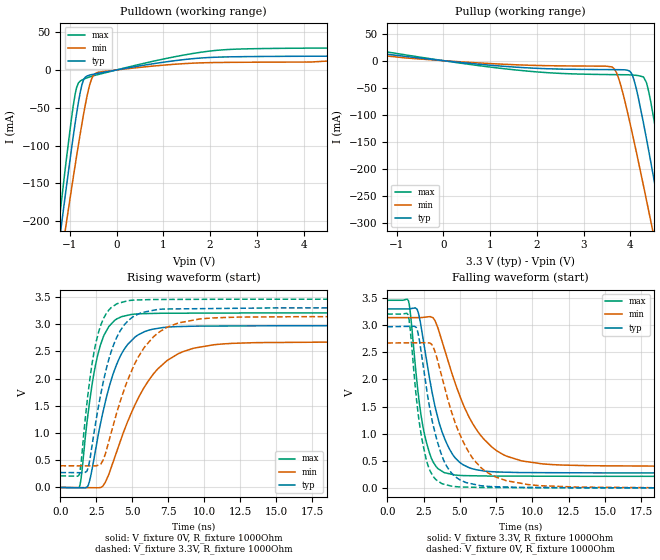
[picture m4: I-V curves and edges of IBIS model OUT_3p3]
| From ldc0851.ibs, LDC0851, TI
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|   Model
[Model]   OUT_3p3
Model_type   Output
Polarity   Non-Inverting
Vmeas = 1.65
Vref = 0
Cref = 1pF
Rref = 100000
|   typ   min   max
C_comp   9.048pF   8.571pF   9.543pF
[Voltage Range]   3.3   3.14   3.46
[Temperature Range]   27   125   -40
[Pullup Reference]   3.3   3.14   3.46
[Pulldown Reference]   0   0   0
[Power Clamp Reference]   3.3   3.14   3.46
[GND Clamp Reference]   0   0   0
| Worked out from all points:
|   slope of the pulldown table from 0 to 0.495 V, typ, clamps not added: 92.7 ohm
|   slope of the pullup table from 0 to 0.495 V, typ, clamps not added: 112 ohm
|   falling waveform, V_fixture 3.3V, R_fixture 1000Ohm: 20-80 % time 1.5ns typ, 2.6ns min, 938ps max; typ from 3.3 V to 0.274 V
|   rising waveform, V_fixture 0V, R_fixture 1000Ohm: 20-80 % time 1.72ns typ, 2.88ns min, 1.1ns max; typ from 0 V to 2.97 V
|   rising waveform, V_fixture 3.3V, R_fixture 1000Ohm: 20-80 % time 1.55ns typ, 2.42ns min, 1.03ns max; typ from 0.274 V to 3.3 V
|   falling waveform, V_fixture 0V, R_fixture 1000Ohm: 20-80 % time 1.36ns typ, 2.24ns min, 888ps max; typ from 2.97 V to 0 V
[Pulldown]
|   Voltage   I(typ)   I(min)   I(max)
-3.3V     -1.297A    -1.195A    -1.39A
-1.29V    -259.5mA   -293.3mA   -234.6mA
-1.191V   -211.2mA   -251.4mA   -180.5mA
-1.082V   -159.1mA   -205.9mA   -122.7mA
-884.4mV  -69.99mA   -125.6mA   -31.72mA
-745.8mV  -21.04mA   -72.9mA    -13.5mA
-567.6mV  -6.71mA    -18.3mA    -9.131mA
-419.1mV  -4.757mA   -3.583mA   -6.489mA
2.095V    16.76mA    9.779mA    25.64mA
5.066V    19.59mA    16.67mA    29.07mA
5.57V     28.17mA    23.1mA     30.75mA
6.6V      47.76mA    36.56mA    53.71mA
[Pullup]
|   Voltage   I(typ)   I(min)   I(max)
-3.3V     47.71mA    34.42mA    57.46mA
-1.944V   21.98mA    16.77mA    26.01mA
432.3mV   -3.873mA   -2.479mA   -5.394mA
3.6V      -16.62mA   -11.54mA   -25.83mA
3.739V    -16.71mA   -30.25mA   -25.95mA
3.937V    -17.62mA   -94.92mA   -26.16mA
4.075V    -35.13mA   -148.5mA   -26.78mA
4.343V    -144mA     -257.9mA   -40.43mA
4.442V    -190.3mA   -299.7mA   -78.92mA
4.63V     -281.3mA   -380.3mA   -174.1mA
4.877V    -404.7mA   -488.4mA   -308.9mA
6.6V      -1.297A    -1.268A    -1.297A
[Ramp]
R_load = 1000
|   typ   min   max
dV/dt_r   1.78296/1.7228e-09   1.60337/2.87484e-09   1.92397/1.09827e-09
dV/dt_f   1.81553/1.49806e-09   1.64494/2.60174e-09   1.94863/9.35822e-10
[Falling Waveform]
V_fixture = 3.3V
V_fixture_min = 3.14V
V_fixture_max = 3.46V
R_fixture = 1000Ohm
C_fixture = 0F
|   Time   V(typ)   V(min)   V(max)
0s        3.3V       3.14V      3.46V
1.452ns   3.3V       3.14V      3.454V
2.051ns   3.296V     3.14V      1.93V
2.467ns   2.745V     3.145V     1.114V
3.057ns   1.805V     3.148V     533.2mV
3.765ns   1.038V     2.709V     307.7mV
4.671ns   554.9mV    1.937V     236.5mV
7.187ns   298.6mV    757.9mV    217.8mV
11.29ns   279.7mV    430.4mV    214.7mV
100ns     274.1mV    398.4mV    212.3mV
[Rising Waveform]
V_fixture = 0V
V_fixture_min = 0V
V_fixture_max = 0V
R_fixture = 1000Ohm
C_fixture = 0F
|   Time   V(typ)   V(min)   V(max)
0s        -209.5nV   -667.8nV   -83.89nV
1.346ns   -5.467mV   -2.915mV   31.72mV
1.894ns   19.73mV    -4.101mV   1.298V
2.409ns   639.4mV    -5.216mV   2.209V
3.016ns   1.45V      51.56mV    2.787V
3.884ns   2.245V     634.7mV    3.09V
4.923ns   2.693V     1.363V     3.178V
7.439ns   2.945V     2.336V     3.201V
11.96ns   2.967V     2.647V     3.205V
100ns     2.972V     2.672V     3.207V
[Rising Waveform]
V_fixture = 3.3V
V_fixture_min = 3.14V
V_fixture_max = 3.46V
R_fixture = 1000Ohm
C_fixture = 0F
|   Time   V(typ)   V(min)   V(max)
0s        274.1mV    398.4mV    212.3mV
1.307ns   271.5mV    397.4mV    233.7mV
1.844ns   300.2mV    397mV      1.549V
2.347ns   1.025V     396.7mV    2.501V
2.816ns   1.726V     432.1mV    2.988V
3.616ns   2.562V     1.086V     3.319V
4.671ns   3.054V     1.969V     3.43V
6.926ns   3.274V     2.864V     3.454V
10.7ns    3.287V     3.116V     3.457V
100ns     3.3V       3.14V      3.46V
[Falling Waveform]
|Gnd
V_fixture = 0V
V_fixture_min = 0V
V_fixture_max = 0V
R_fixture = 1000Ohm
C_fixture = 0F
|   Time   V(typ)   V(min)   V(max)
0s        2.972V     2.672V     3.207V
1.429ns   2.979V     2.675V     3.195V
2.006ns   2.954V     2.676V     1.649V
2.409ns   2.368V     2.677V     865.7mV
2.938ns   1.45V      2.671V     319.1mV
3.659ns   670.8mV    2.152V     96.29mV
4.451ns   267.8mV    1.381V     29.94mV
6.65ns    33.68mV    329.8mV    6.918mV
10.7ns    6.35mV     37.61mV    2.916mV
100ns     -209.5nV   -667nV     -87.55nV
